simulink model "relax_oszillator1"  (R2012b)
settings: Solver=ode45  StartTime=0.0  StopTime=100.0  MaxStep=0.01  RelTol=1e-3
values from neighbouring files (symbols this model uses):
  Th = 1    [fuellstnd_3.m]    (also in fuellstnd_31.m; regulator_1.m = 10; zweipunkt_31.m = 100; zweipunkt_32.m = 100)
  Tp = 1    [fuellstnd_2.m]    (also in fuellstnd_21.m = 0.1; fuellstnd_3.m = 0.1; fuellstnd_31.m = 0.01; regulator_1.m = 5)
libraries: dspstat3 x1

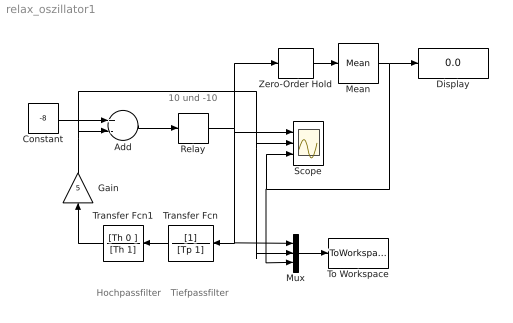
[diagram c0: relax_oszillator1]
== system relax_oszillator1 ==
  note: Hochpassfilter
  note: Tiefpassfilter
  note: 10 und -10
  Add : Sum  Inputs=+-
  Constant : Constant  Value=-8
  Display : Display
  Gain : Gain  Gain=5
  Mean : dspstat3/Mean  run=on  reset_popup=None  InputProcessing=Columns as channels (frame based)  directionMode=Each column  dimension=1  treatSBRowAsCol=on  roiEnable=off  roiType=Rectangles  roiPortion=Entire ROI  roiOutput=Individual statistics for each ROI  roiFlag=off  outputDataTypeStr=Inherit: Same as accumulator  outputLastDataTypeStr=Inherit: Same as accumulator  outputMin=[]  outputMax=[]  roundingMode=Floor  overflowMode=off
  Mux : Mux  Inputs=3
  Relay : Relay  OnSwitchValue=1  OffSwitchValue=-1  OnOutputValue=20  OffOutputValue=-20
  Scope : Scope  NumInputPorts=3
  To Workspace : ToWorkspace  VariableName=y  SampleTime=-1  SaveFormat=Structure With Time
  Transfer Fcn : TransferFcn  Denominator=[Tp 1]
  Transfer Fcn1 : TransferFcn  Numerator=[Th 0 ]  Denominator=[Th 1]
  Zero-Order Hold : ZeroOrderHold  SampleTime=0.01
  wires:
  Add/1 -> Relay/1
  Relay/1 -> Zero-Order Hold/1, Mux/1, Transfer Fcn/1, Scope/1
  Constant/1 -> Add/1
  Mean/1 -> Mux/3, Scope/3, Display/1
  Zero-Order Hold/1 -> Mean/1
  Mux/1 -> To Workspace/1
  Gain/1 -> Add/2, Mux/2, Scope/2
  Transfer Fcn/1 -> Transfer Fcn1/1
  Transfer Fcn1/1 -> Gain/1
